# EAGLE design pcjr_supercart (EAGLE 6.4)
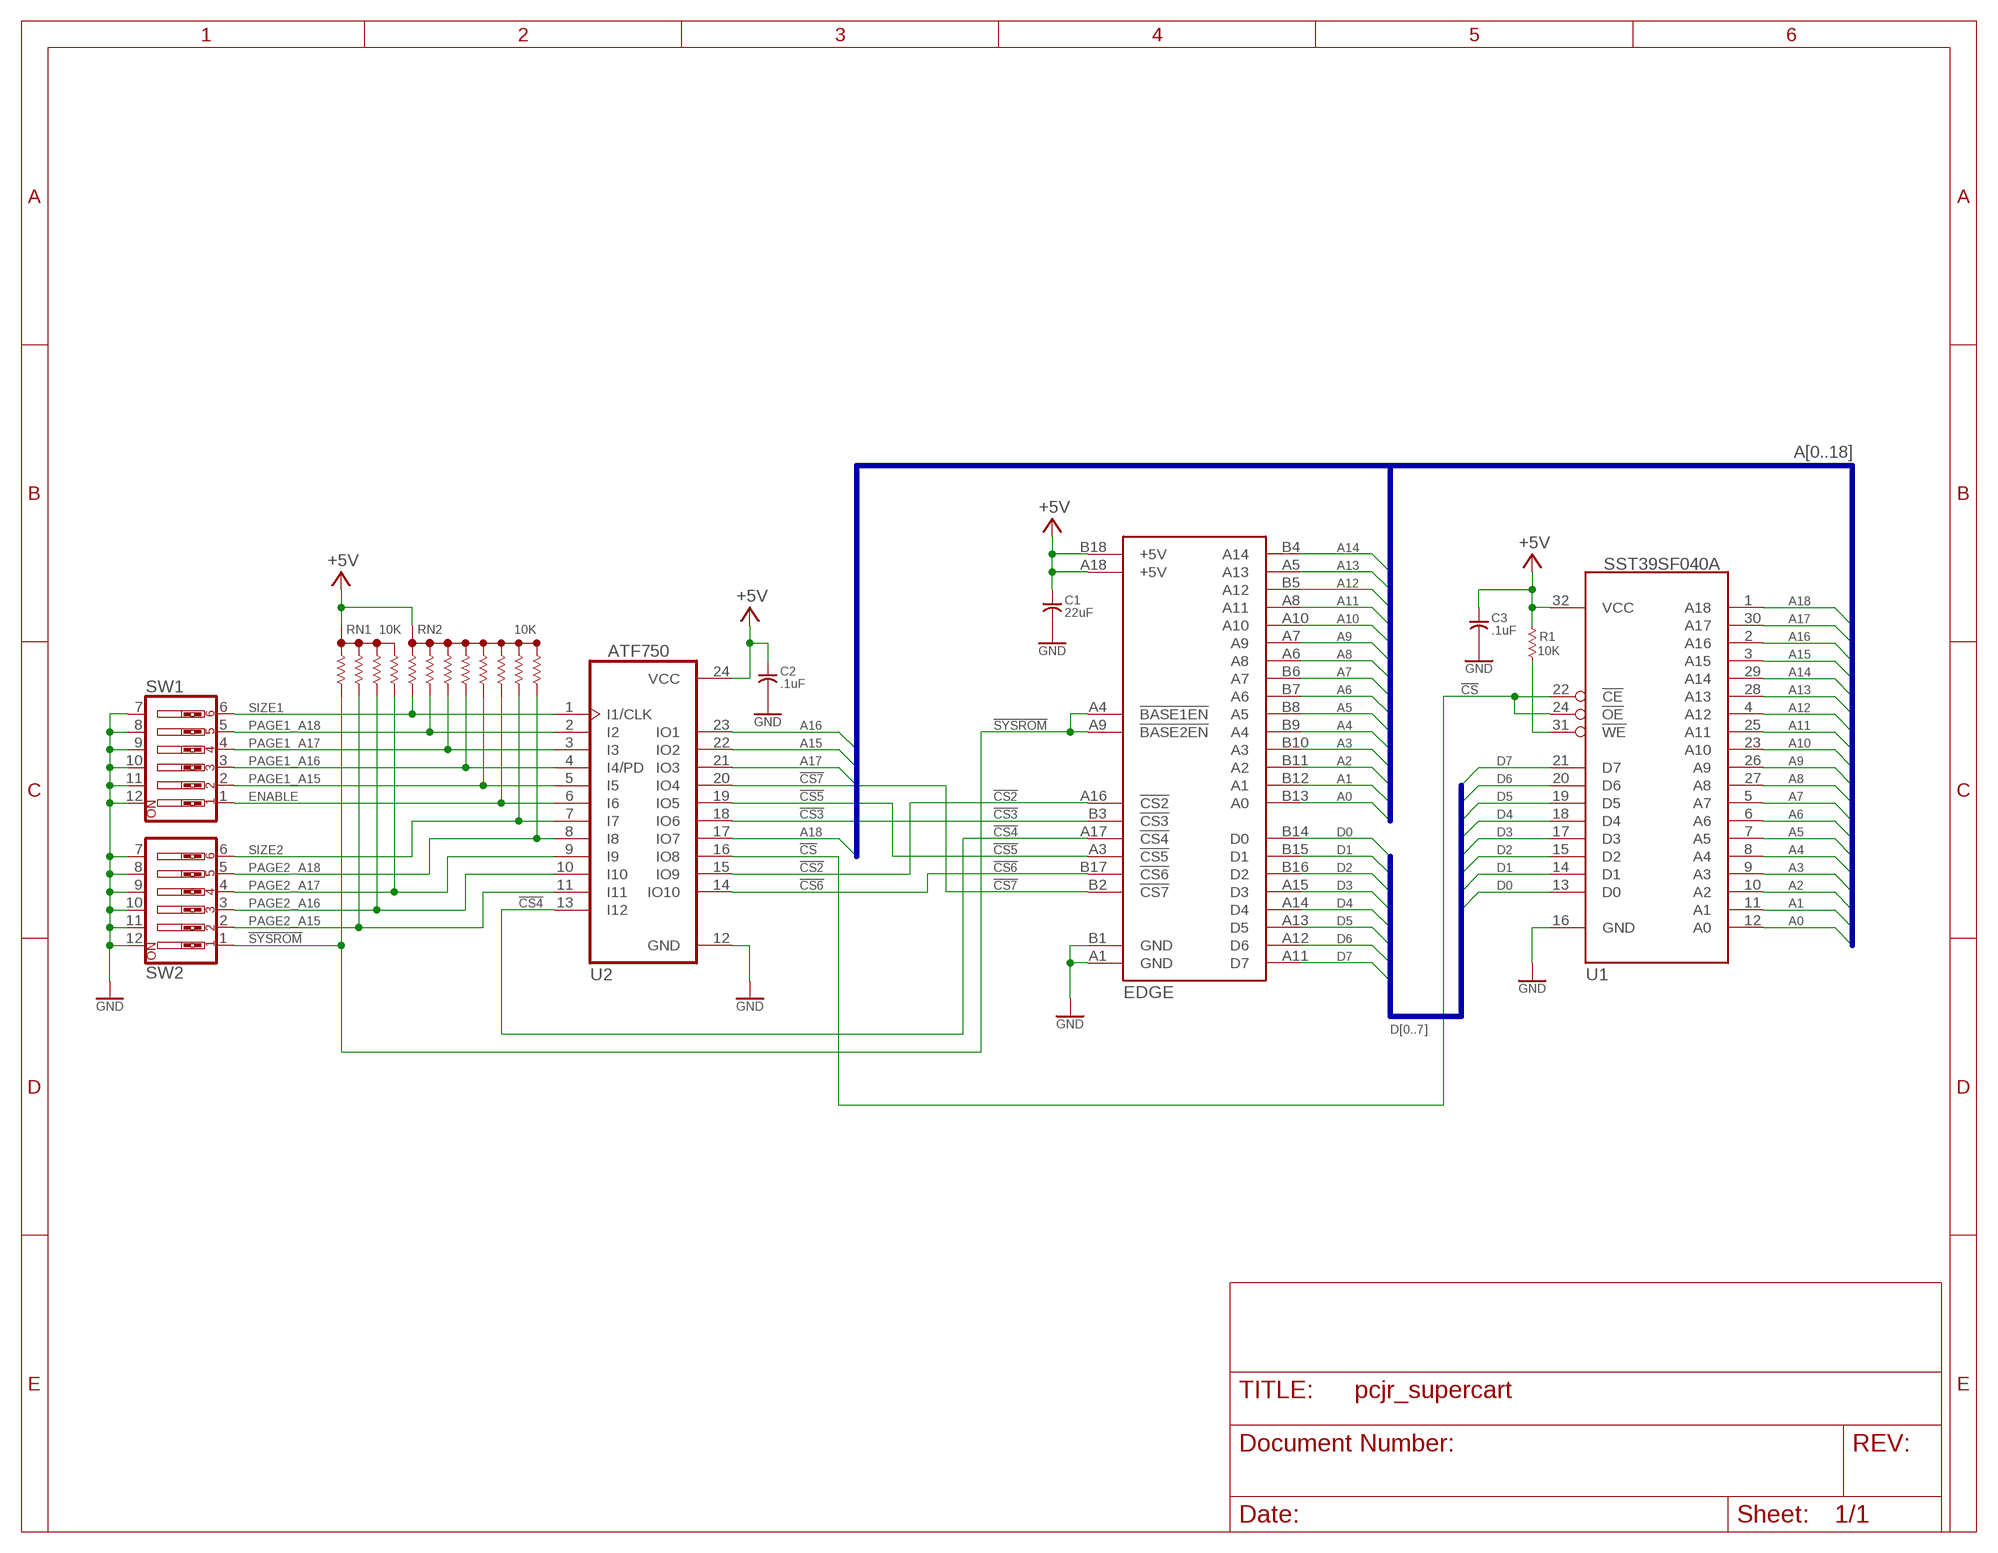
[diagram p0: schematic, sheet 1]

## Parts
C1  22uF  C_US  [C_TH_5MM]
C2  .1uF  C_US  [C_TH_5MM]
C3  .1uF  C_US  [C_TH_5MM]
EDGE  PCJR_CARTRIDGE  [PCJR_CARTRIDGE]
R1  10K  R_US  [R_204/7]
RN1  10K  RNET_X4  [RN_SIP5]
RN2  10K  RNET_X8_SIP  [RN_SIP9]
SW1  SW_DIP-6  [SW_DIP-6]
SW2  SW_DIP-6  [SW_DIP-6]
U1  SST39SF040A  [DIL32W]
U2  ATF750  22V10P  [DIL24]

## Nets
!CS: U1.22(!CE) U1.24(!OE) U2.16(IO8)
!CS2: EDGE.A16(!CS2) U2.15(IO9)
!CS3: EDGE.B3(!CS3) U2.18(IO6)
!CS4: EDGE.A17(!CS4) U2.13(I12)
!CS5: EDGE.A3(!CS5) U2.19(IO5)
!CS6: EDGE.B17(!CS6) U2.14(IO10)
!CS7: EDGE.B2(!CS7) U2.20(IO4)
!SYSROM: EDGE.A4(!BASE1EN) EDGE.A9(!BASE2EN) RN1.2 SW2.1
+5V: C1.1 C2.1 C3.1 EDGE.A18(+5V) EDGE.B18(+5V) R1.2 RN1.1 RN2.1 U1.32(VCC) U2.24(VCC)
A0: EDGE.B13(A0) U1.12(A0)
A1: EDGE.B12(A1) U1.11(A1)
A2: EDGE.B11(A2) U1.10(A2)
A3: EDGE.B10(A3) U1.9(A3)
A4: EDGE.B9(A4) U1.8(A4)
A5: EDGE.B8(A5) U1.7(A5)
A6: EDGE.B7(A6) U1.6(A6)
A7: EDGE.B6(A7) U1.5(A7)
A8: EDGE.A6(A8) U1.27(A8)
A9: EDGE.A7(A9) U1.26(A9)
A10: EDGE.A10 U1.23(A10)
A11: EDGE.A8(A11) U1.25(A11)
A12: EDGE.B5(A12) U1.4(A12)
A13: EDGE.A5(A13) U1.28(A13)
A14: EDGE.B4(A14) U1.29(A14)
A15: U1.3(A15) U2.22(IO2)
A16: U1.2(A16) U2.23(IO1)
A17: U1.30(A17) U2.21(IO3)
A18: U1.1(A18) U2.17(IO7)
D0: EDGE.B14(D0) U1.13(D0)
D1: EDGE.B15(D1) U1.14(D1)
D2: EDGE.B16(D2) U1.15(D2)
D3: EDGE.A15(D3) U1.17(D3)
D4: EDGE.A14(D4) U1.18(D4)
D5: EDGE.A13(D5) U1.19(D5)
D6: EDGE.A12(D6) U1.20(D6)
D7: EDGE.A11(D7) U1.21(D7)
ENABLE: RN2.7 SW1.1 U2.6(I6)
GND: C1.2 C2.2 C3.2 EDGE.A1(GND) EDGE.B1(GND) SW1.7 SW1.8 SW1.9 SW1.10 SW1.11 SW1.12 SW2.7 SW2.8 SW2.9 SW2.10 SW2.11 SW2.12 U1.16(GND) U2.12(GND)
N$10: R1.1 U1.31(!WE)
PAGE1_A15: RN2.6 SW1.2 U2.5(I5)
PAGE1_A16: RN2.5 SW1.3 U2.4(I4/PD)
PAGE1_A17: RN2.4 SW1.4 U2.3(I3)
PAGE1_A18: RN2.3 SW1.5 U2.2(I2)
PAGE2_A15: RN1.3 SW2.2 U2.11(I11)
PAGE2_A16: RN1.4 SW2.3 U2.10(I10)
PAGE2_A17: RN1.5 SW2.4 U2.9(I9)
PAGE2_A18: RN2.9 SW2.5 U2.8(I8)
SIZE1: RN2.2 SW1.6 U2.1(I1/CLK)
SIZE2: RN2.8 SW2.6 U2.7(I7)

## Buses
A[0..18]
D[0..7]

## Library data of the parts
C1-C3 = alan_common:C_US
EDGE = alan_common:PCJR_CARTRIDGE
R1 = alan_common:R_US
RN1 = alan_common:RNET_X4
RN2 = alan_common:RNET_X8_SIP
SW1 SW2 = alan_common:SW_DIP-6
U1 = alan_common:SST39SF040A: 4MB 5V Flash JEDEC
U2 = alan_common:22V10

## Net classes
0 default: width 0.254 mm, drill 0.33 mm, clearance 0.203 mm

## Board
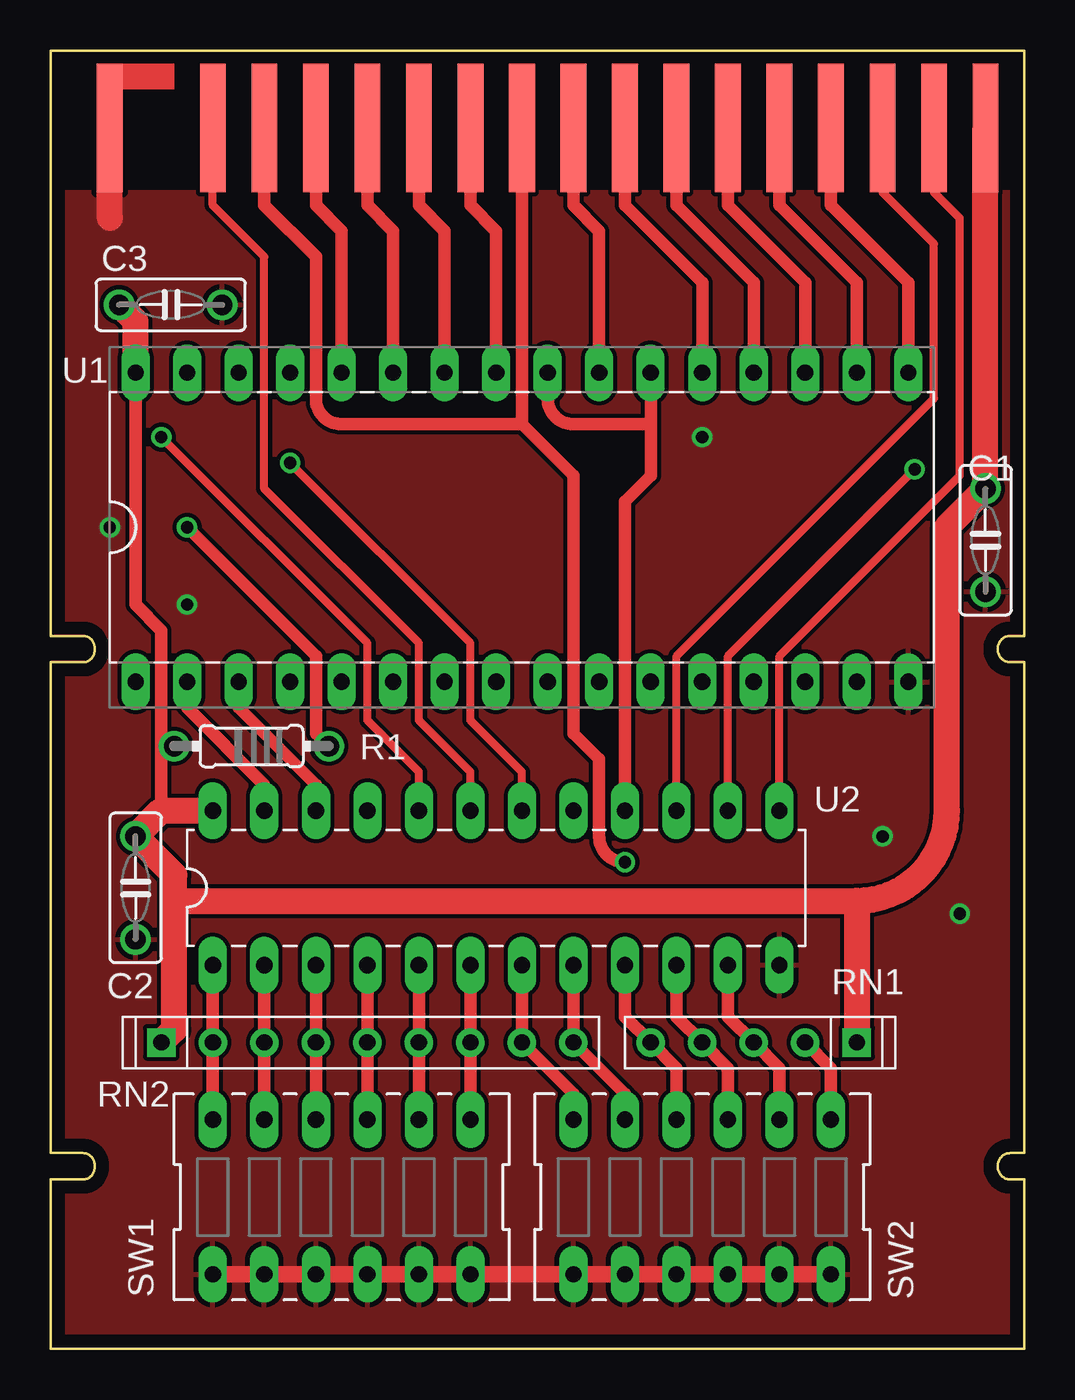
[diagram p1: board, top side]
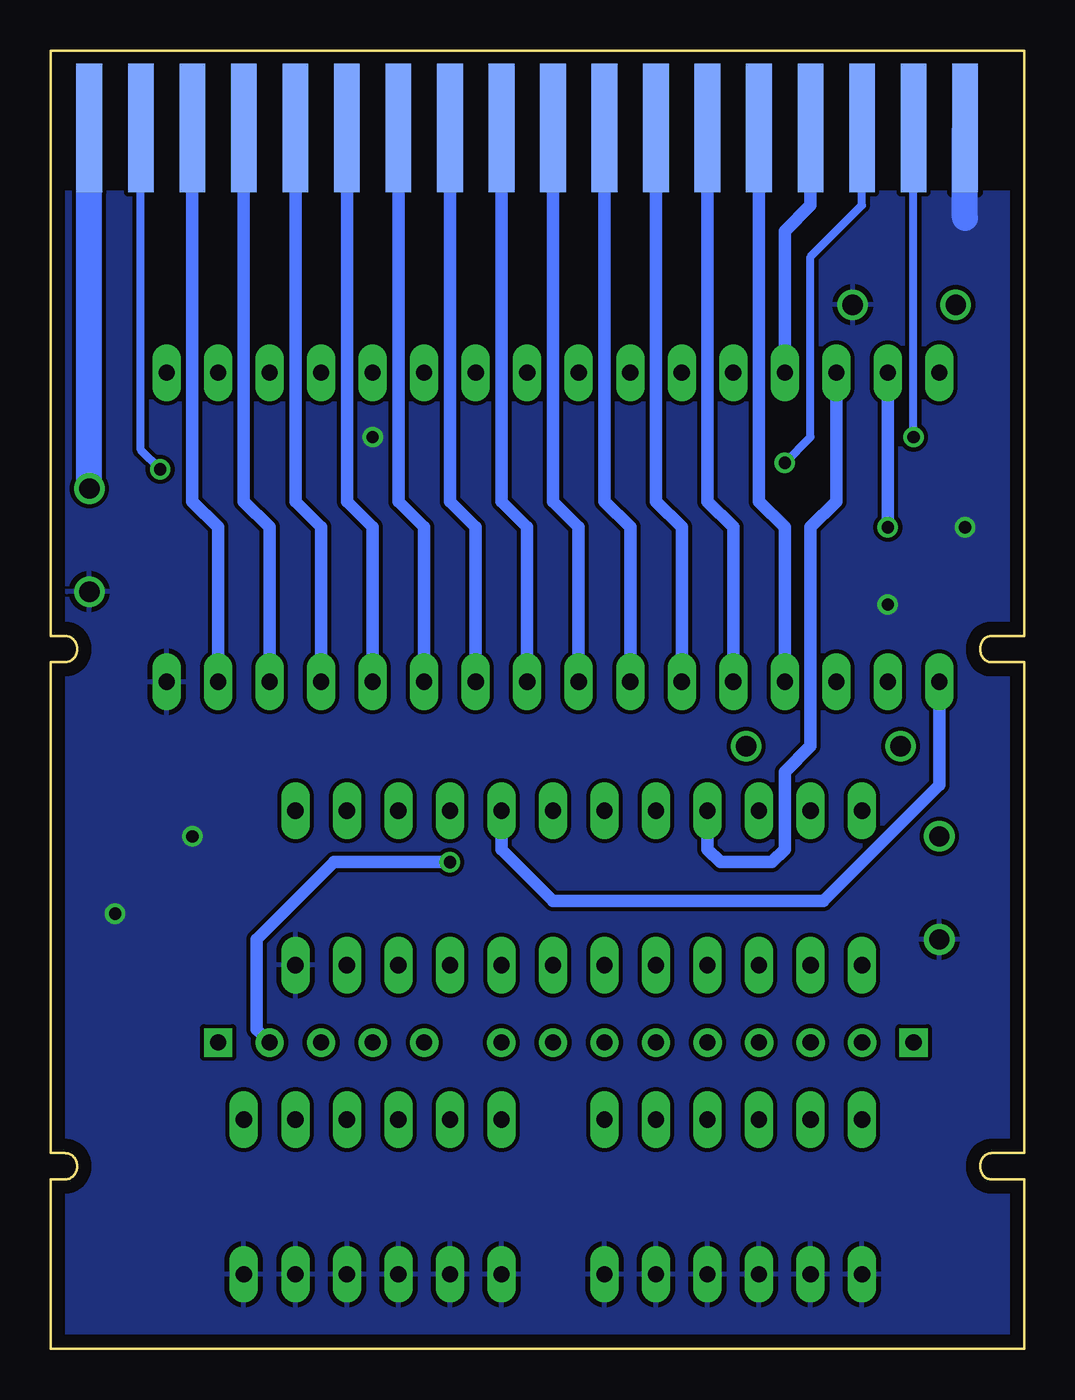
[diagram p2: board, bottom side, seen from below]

Size 48 x 64 mm. Coordinates in mm from the lower left corner, seen from the top.
Copper layers (1*16): Top 0.035mm / dielectric 1.5mm / Bottom 0.035mm
Design rules "default": minimum track width 10mil, minimum drill 13mil, track to track 8mil, track to pad 8mil, pad to pad 8mil, via to via 8mil, smd to smd 8mil, copper to edge 25mil, drill to drill 8mil, minimum pad ring 10mil, minimum via ring 8mil, stop-mask expansion 4mil, vias tented up to drill 0mil, thermal gap 10mil

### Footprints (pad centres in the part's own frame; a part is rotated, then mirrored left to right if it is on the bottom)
C_TH_5MM = drill 1: 1 -2.54,0; 2 2.54,0
PCJR_CARTRIDGE = smd 1.27 x 6.35: A1 45.085,3.81; A3 40.005,3.81; A4 37.465,3.81; A5 34.925,3.81; A6 32.385,3.81; A7 29.845,3.81; A8 27.305,3.81; A9 24.765,3.81; A10 22.225,3.81; A11 19.685,3.81; A12 17.145,3.81; A13 14.605,3.81; A14 12.065,3.81; A15 9.525,3.81; A16 6.985,3.81; A17 4.445,3.81; A18 1.905,3.81 | smd 1.27 x 6.35 bottom: B1 45.085,3.81; B2 42.545,3.81; B3 40.005,3.81; B4 37.465,3.81; B5 34.925,3.81; B6 32.385,3.81; B7 29.845,3.81; B8 27.305,3.81; B9 24.765,3.81; B10 22.225,3.81; B11 19.685,3.81; B12 17.145,3.81; B13 14.605,3.81; B14 12.065,3.81; B15 9.525,3.81; B16 6.985,3.81; B17 4.445,3.81; B18 1.905,3.81
R_204/7 = drill 1: 1 -3.81,0; 2 3.81,0
RN_SIP5 = drill 0.8 pad 1.4 square: 1 -5.08,0 | drill 0.8 pad 1.4: 2 -2.54,0; 3 0,0; 4 2.54,0; 5 5.08,0
RN_SIP9 = drill 0.8 pad 1.4 square: 1 -10.16,0 | drill 0.8 pad 1.4: 2 -7.62,0; 3 -5.08,0; 4 -2.54,0; 5 0,0; 6 2.54,0; 7 5.08,0; 8 7.62,0; 9 10.16,0
SW_DIP-6 = drill 0.8 pad 1.4 long: 1 -6.35,-3.81; 2 -3.81,-3.81; 3 -1.27,-3.81; 4 1.27,-3.81; 5 3.81,-3.81; 6 6.35,-3.81; 7 6.35,3.81; 8 3.81,3.81; 9 1.27,3.81; 10 -1.27,3.81; 11 -3.81,3.81; 12 -6.35,3.81
DIL32W = drill 0.8 pad 1.4 long: 1 -21.59,-7.62; 2 -19.05,-7.62; 3 -16.51,-7.62; 4 -13.97,-7.62; 5 -11.43,-7.62; 6 -8.89,-7.62; 7 -6.35,-7.62; 8 -3.81,-7.62; 9 -1.27,-7.62; 10 1.27,-7.62; 11 3.81,-7.62; 12 6.35,-7.62; 13 8.89,-7.62; 14 11.43,-7.62; 15 13.97,-7.62; 16 16.51,-7.62; 17 16.51,7.62; 18 13.97,7.62; 19 11.43,7.62; 20 8.89,7.62; 21 6.35,7.62; 22 3.81,7.62; 23 1.27,7.62; 24 -1.27,7.62; 25 -3.81,7.62; 26 -6.35,7.62; 27 -8.89,7.62; 28 -11.43,7.62; 29 -13.97,7.62; 30 -16.51,7.62; 31 -19.05,7.62; 32 -21.59,7.62
DIL24 = drill 0.8 pad 1.4 long: 1 -10.16,-3.81; 2 -7.62,-3.81; 3 -5.08,-3.81; 4 -2.54,-3.81; 5 0,-3.81; 6 2.54,-3.81; 7 5.08,-3.81; 8 7.62,-3.81; 9 10.16,-3.81; 10 12.7,-3.81; 11 15.24,-3.81; 12 17.78,-3.81; 13 17.78,3.81; 14 15.24,3.81; 15 12.7,3.81; 16 10.16,3.81; 17 7.62,3.81; 18 5.08,3.81; 19 2.54,3.81; 20 0,3.81; 21 -2.54,3.81; 22 -5.08,3.81; 23 -7.62,3.81; 24 -10.16,3.81

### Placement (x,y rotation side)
C1  46.09,39.87 270 top
C2  4.18,22.73 270 top
C3  5.92,51.48 0 top
EDGE  48,64 180 top
R1  9.9,29.71 180 top
RN1  34.66,15.11 180 top
RN2  15.62,15.11 0 top
SW1  14.35,7.49 180 top
SW2  32.12,7.49 180 top
U1  25.77,40.51 0 top
U2  18.16,22.73 0 top

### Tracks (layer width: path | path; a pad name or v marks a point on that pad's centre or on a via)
!CS
  Top 0.61: U1.24 24.5,46.85 arc90 25.77,45.59 29.59,45.59 | 29.59,45.59 U1.22 | 29.59,45.59 29.59,43.05 28.32,41.77 U2.16
!CS2
  Top 0.406: EDGE.A16 41.02,57.02 43.55,54.48 43.55,46.85 30.86,34.16 U2.15
!CS3  (via drill 0.6)
  Top 0.406: U2.18 23.23,28.44 20.7,30.98 20.7,34.79 v11.8,43.68
  Bottom 0.406: EDGE.B3 8,56.38 10.54,53.84 10.54,44.95 v11.8,43.68
!CS4
  Top 0.406: EDGE.A17 43.55,57.02 44.83,55.74 44.83,43.05 35.94,34.16 U2.13
!CS5
  Top 0.406: EDGE.A3 8,56.38 10.54,53.84 10.54,42.41 18.16,34.79 18.16,30.98 20.7,28.44 U2.19
!CS6  (via drill 0.6)
  Top 0.406: U2.14 33.4,34.16 v42.6,43.36
  Bottom 0.406: EDGE.B17 43.55,44.31 v42.6,43.36
!CS7  (via drill 0.6)
  Top 0.406: U2.20 18.16,28.44 15.62,30.98 15.62,34.79 v5.46,44.95
  Bottom 0.406: v5.46,44.95 EDGE.B2
!SYSROM  (via drill 0.6)
  Top 0.61: EDGE.A4 10.54,56.38 13.07,53.84 13.07,46.85 arc90 14.35,45.59 23.23,45.59 | SW2.1 38.48,13.84 RN1.2 | v28.32,24 arc-90 27.05,25.27 27.05,29.07 25.77,30.34 25.77,43.05 23.23,45.59 | 23.23,45.59 EDGE.A9
  Bottom 0.61: RN1.2 37.84,15.74 37.84,20.18 34.03,24 v28.32,24
+5V
  Top 0.61: 5.46,26.54 5.46,29.71 | 5.46,29.71 5.46,35.42 4.18,36.7 U1.32 | 5.46,29.71 R1.2
  Top 1.27: U2.24 5.46,26.54 C2.1 6.09,23.36 6.09,22.09 | 6.09,22.09 6.09,15.74 RN2.1 | EDGE.A18 C1.1 44.19,40.51 44.19,26.54 arc-90 39.74,22.09 | 6.09,22.09 39.74,22.09 | 39.74,22.09 RN1.1 | U1.32 4.18,50.66 C3.1
  Bottom 1.27: C1.1 EDGE.A18
A0
  Bottom 0.61: EDGE.B13 33.4,41.77 32.12,40.51 U1.12
A1
  Bottom 0.61: EDGE.B12 30.86,41.77 29.59,40.51 U1.11
A2
  Bottom 0.61: EDGE.B11 28.32,41.77 27.05,40.51 U1.10
A3
  Bottom 0.61: EDGE.B10 25.77,41.77 24.5,40.51 U1.9
A4
  Bottom 0.61: EDGE.B9 23.23,41.77 21.96,40.51 U1.8
A5
  Bottom 0.61: EDGE.B8 20.7,41.77 19.43,40.51 U1.7
A6
  Bottom 0.61: EDGE.B7 18.16,41.77 16.89,40.51 U1.6
A7
  Bottom 0.61: EDGE.B6 15.62,41.77 14.35,40.51 U1.5
A8
  Top 0.61: EDGE.A6 15.62,56.38 16.89,55.11 U1.27
A9
  Top 0.61: EDGE.A7 18.16,56.38 19.43,55.11 U1.26
A10
  Top 0.61: EDGE.A10 25.77,56.38 27.05,55.11 U1.23
A11
  Top 0.61: EDGE.A8 20.7,56.38 21.96,55.11 U1.25
A12
  Bottom 0.61: EDGE.B5 13.07,41.77 11.8,40.51 U1.4
A13
  Top 0.61: EDGE.A5 13.07,56.38 14.35,55.11 U1.28
A14
  Bottom 0.61: EDGE.B4 10.54,56.38 11.8,55.11 U1.29
A15
  Top 0.61: U1.3 9.27,31.61 13.07,27.8 U2.22
A16
  Top 0.61: U1.2 6.72,31.61 10.54,27.8 U2.23
A17
  Bottom 0.61: U1.30 9.27,41.77 10.54,40.51 10.54,29.71 11.8,28.44 11.8,24.63 12.44,24 14.98,24 15.62,24.63 U2.21
A18
  Bottom 0.61: U1.1 4.18,27.8 9.9,22.09 23.23,22.09 25.77,24.63 U2.17
D0
  Bottom 0.61: EDGE.B14 35.94,41.77 34.66,40.51 U1.13
D1
  Bottom 0.61: EDGE.B15 38.48,41.77 37.2,40.51 U1.14
D2
  Bottom 0.61: EDGE.B16 41.02,41.77 39.74,40.51 U1.15
D3
  Top 0.61: EDGE.A15 38.48,56.38 42.28,52.57 U1.17
D4
  Top 0.61: EDGE.A14 35.94,56.38 39.74,52.57 U1.18
D5
  Top 0.61: EDGE.A13 33.4,56.38 37.2,52.57 U1.19
D6
  Top 0.61: EDGE.A12 30.86,56.38 34.66,52.57 U1.20
D7
  Top 0.61: EDGE.A11 28.32,56.38 32.12,52.57 U1.21
ENABLE
  Top 0.61: SW1.1 RN2.7 U2.6
GND  (via drill 0.6)
  Top 0.813: SW2.12 SW2.11 SW2.10 SW2.9 SW2.8 SW2.7 SW1.12 SW1.11 SW1.10 SW1.9 SW1.8 SW1.7
  Top 1.27: 2.92,55.74 EDGE.A1
  Bottom 1.27: 2.92,55.74 EDGE.A1
  other vias: 6.72,36.7 2.92,40.51 44.83,21.45 41.02,25.27 32.12,44.95
  pour Top: 48,0 48,57 0,57 0,0
  pour Bottom: 48,0 48,57 0,57 0,0
N$10  (via drill 0.6)
  Top 0.61: R1.1 13.07,30.34 13.07,34.16 v6.72,40.51
  Bottom 0.61: v6.72,40.51 U1.31
PAGE1_A15
  Top 0.61: SW1.2 RN2.6 U2.5
PAGE1_A16
  Top 0.61: SW1.3 RN2.5 U2.4
PAGE1_A17
  Top 0.61: SW1.4 RN2.4 U2.3
PAGE1_A18
  Top 0.61: SW1.5 RN2.3 U2.2
PAGE2_A15
  Top 0.61: SW2.2 35.94,13.84 RN1.3 33.4,16.38 U2.11
PAGE2_A16
  Top 0.61: SW2.3 33.4,13.84 RN1.4 30.86,16.38 U2.10
PAGE2_A17
  Top 0.61: SW2.4 30.86,13.84 RN1.5 28.32,16.38 U2.9
PAGE2_A18
  Top 0.61: SW2.5 28.32,12.56 RN2.9 U2.8
SIZE1
  Top 0.61: SW1.6 RN2.2 U2.1
SIZE2
  Top 0.61: SW2.6 25.77,12.56 RN2.8 U2.7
